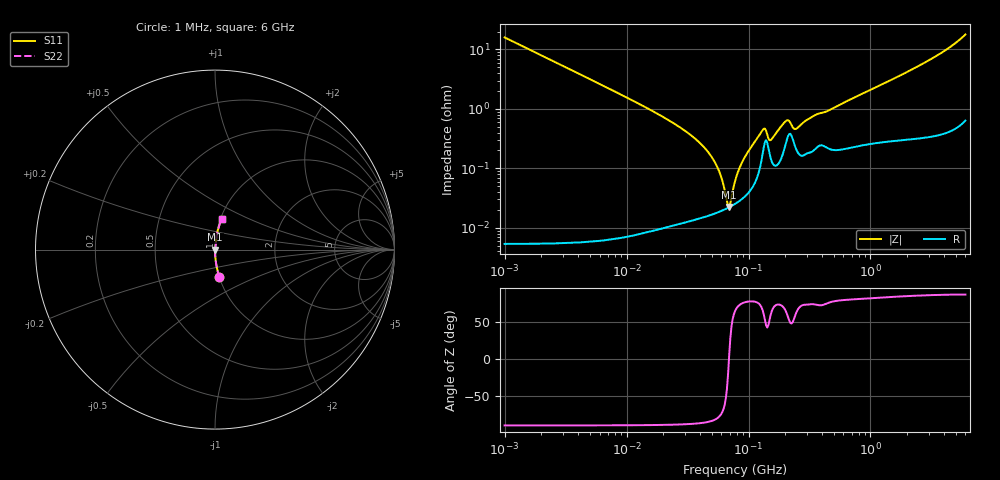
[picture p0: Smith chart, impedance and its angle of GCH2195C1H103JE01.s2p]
!Murata Part Number: GCH2195C1H103JE01
!These Parameters are Measured in Series Mode Connection
!Data Generated on Jun 19, 2026
!  o--ll--o
!Port1  Port2
!  o------o
!Operation Temp=25[degC], DC Bias Voltage=0[V]
!Freq. Start=1000[kHz] Stop=6[GHz] 401[Steps]
# Hz S RI R 50
!Freq.(Hz) S11(Real) S11(Imag) S21(Real) S21(Imag) S12(Real) S12(Imag) S22(Real) S22(Imag)
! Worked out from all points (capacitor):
!   401 points, 1 MHz to 6 GHz, reference 50 ohm
!   read as one part in series: C = 9.99 nF near 1.044 MHz
!   lowest |Z| = 22.3 mohm at 69.48 MHz (marker M1)
!   series resonance near 69.11 MHz, so ESL is about 530 pH
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1000000  0.0248 -0.1553  0.9752 0.1553  0.9752 0.1553  0.0248 -0.1553
4293785  0.00142 -0.0369  0.9986 0.0369  0.9986 0.0369  0.00142 -0.0369
1.843659e7  0.000158 -0.00801  0.9998 0.00801  0.9998 0.00801  0.000158 -0.00801
3.245342e7  0.000142 -0.00382  0.9999 0.00382  0.9999 0.00382  0.000142 -0.00382
4.596069e7  0.000161 -0.00194  0.9998 0.00194  0.9998 0.00194  0.000161 -0.00194
5.589783e7  0.000182 -0.000998  0.9998 0.000998  0.9998 0.000998  0.000182 -0.000998
6.097846e7  0.000196 -0.000589  0.9998 0.000589  0.9998 0.000589  0.000196 -0.000589
6.652088e7  0.000212 -0.00018  0.9998 0.00018  0.9998 0.00018  0.000212 -0.00018
6.947823e7  0.000222 2.55e-05  0.9998 -2.55e-05  0.9998 -2.55e-05  0.000222 2.55e-05
7.256705e7  0.000233 0.000233  0.9998 -0.000233  0.9998 -0.000233  0.000233 0.000233
7.745967e7  0.000252 0.000548  0.9997 -0.000548  0.9997 -0.000548  0.000252 0.000548
8.268215e7  0.000276 0.000872  0.9997 -0.000872  0.9997 -0.000872  0.000276 0.000872
9.218041e7  0.00033 0.00144  0.9997 -0.00144  0.9997 -0.00144  0.00033 0.00144
1.305463e8  0.00176 0.00404  0.9982 -0.00404  0.9982 -0.00404  0.00176 0.00404
1.363501e8  0.00278 0.0037  0.9972 -0.0037  0.9972 -0.0037  0.00278 0.0037
1.520136e8  0.00147 0.00259  0.9985 -0.00259  0.9985 -0.00259  0.00147 0.00259
2.016844e8  0.00258 0.00563  0.9974 -0.00563  0.9974 -0.00563  0.00258 0.00563
2.452905e8  0.00213 0.00408  0.9979 -0.00408  0.9979 -0.00408  0.00213 0.00408
3.325952e8  0.00196 0.00709  0.998 -0.00709  0.998 -0.00709  0.00196 0.00709
1.428092e9  0.00368 0.0293  0.9963 -0.0293  0.9963 -0.0293  0.00368 0.0293
3.408564e9  0.00918 0.0751  0.9908 -0.0751  0.9908 -0.0751  0.00918 0.0751
6e9  0.0366 0.1707  0.9634 -0.1707  0.9634 -0.1707  0.0366 0.1707
